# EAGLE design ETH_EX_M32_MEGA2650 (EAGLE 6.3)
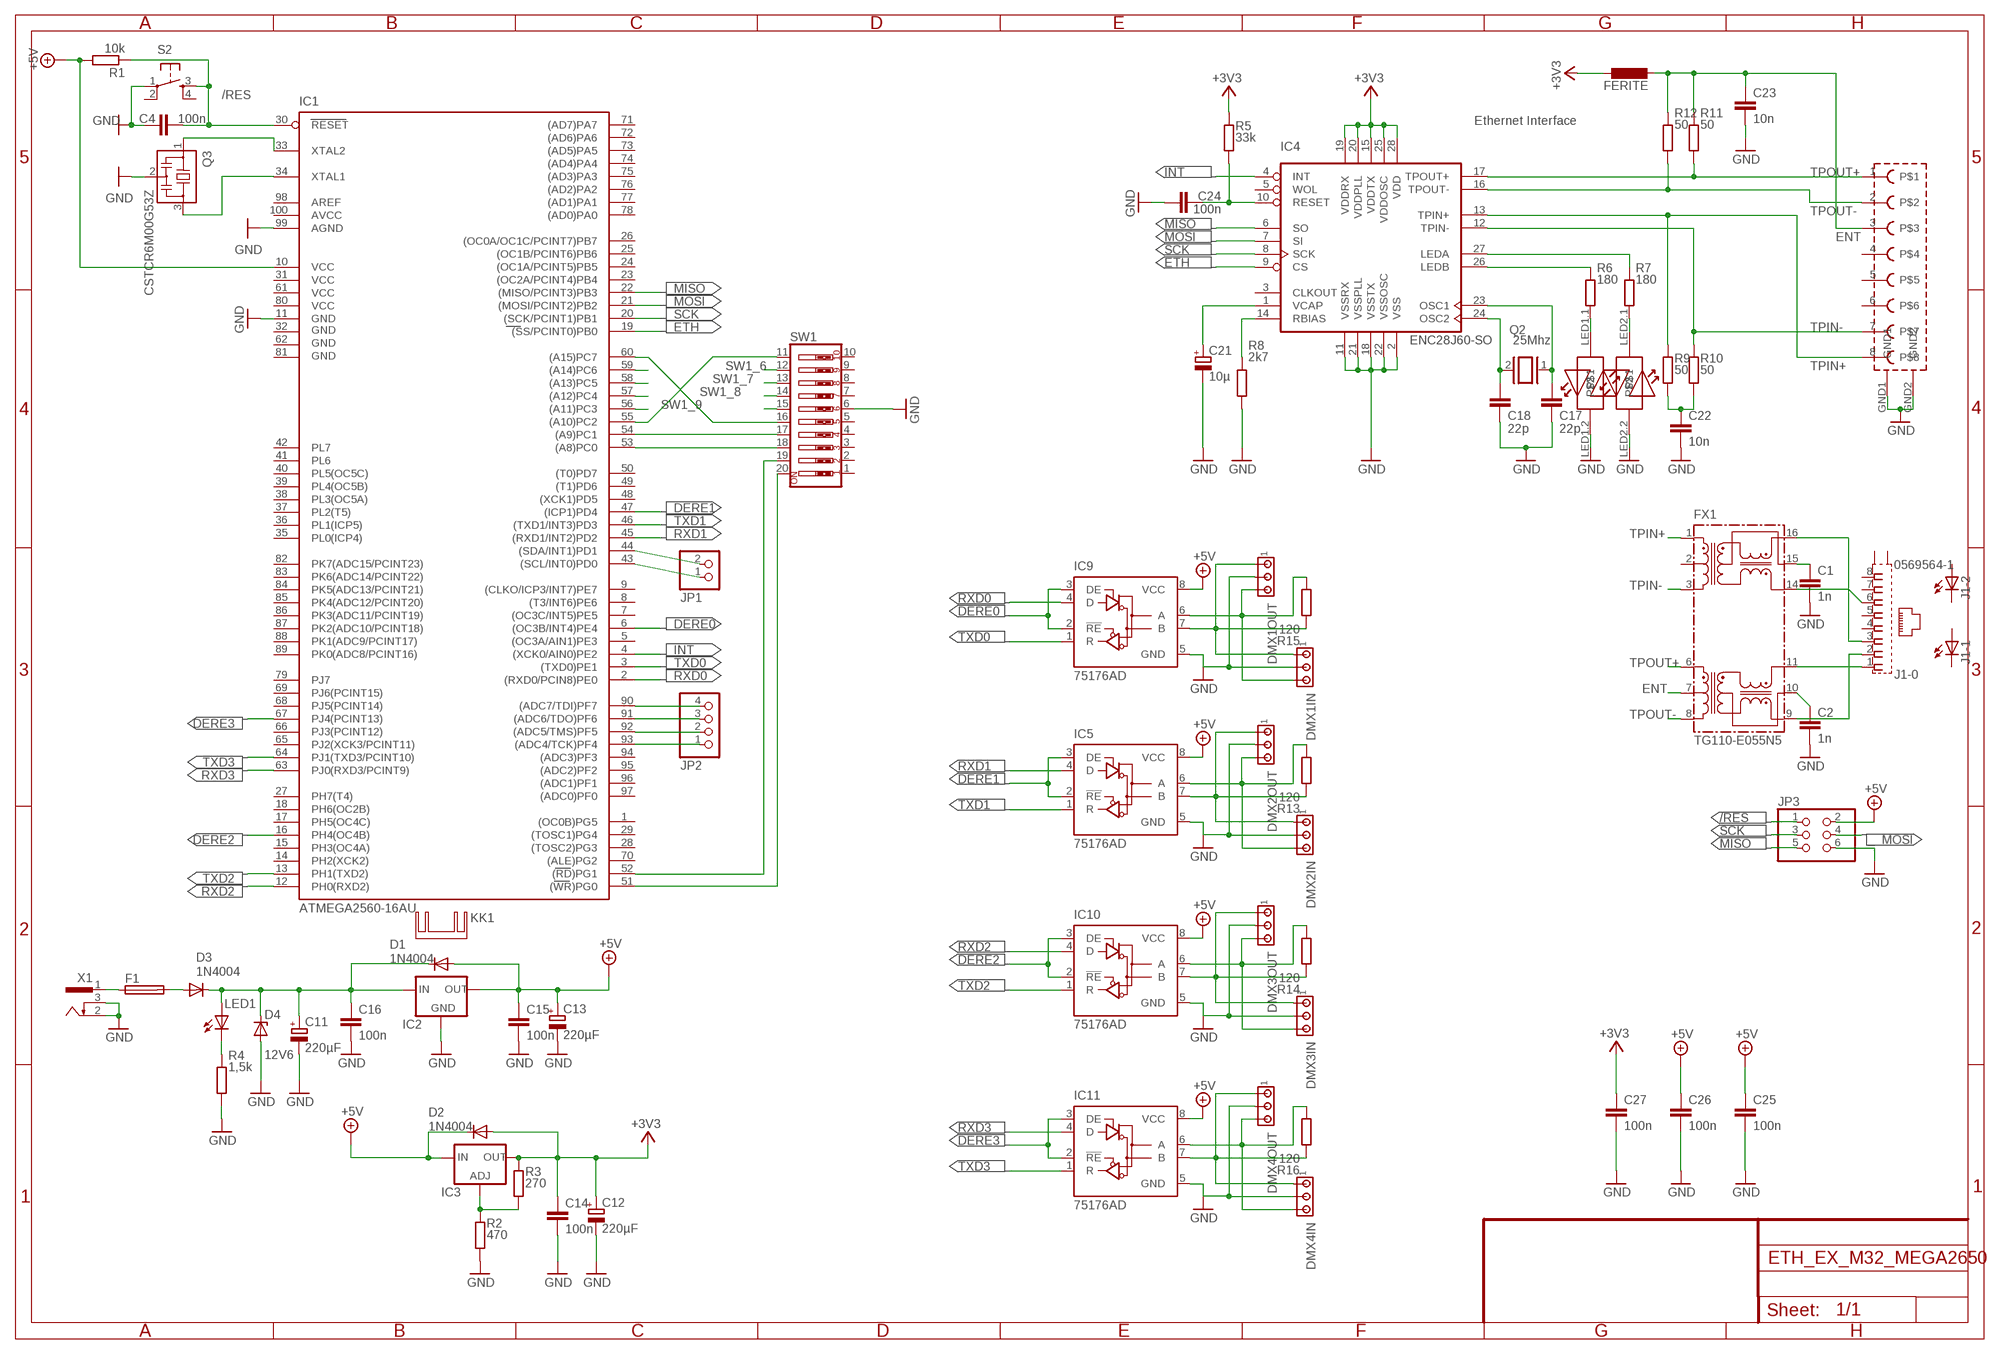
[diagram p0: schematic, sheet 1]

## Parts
C1  1n  C-EUC0805K  [C0805K]
C2  1n  C-EUC0805K  [C0805K]
C4  100n  C-EUC0805K  [C0805K]
C11  220µF  CPOL-EUE3.5-8  [E3,5-8]
C12  220µF  CPOL-EUE3.5-8  [E3,5-8]
C13  220µF  CPOL-EUE3.5-8  [E3,5-8]
C14  100n  C-EU025-024X044  [C025-024X044]
C15  100n  C-EU050-024X044  [C050-024X044]
C16  100n  C-EU050-024X044  [C050-024X044]
C17  22p  C-EUC0805K  [C0805K]
C18  22p  C-EUC0805K  [C0805K]
C21  10µ  CPOL-EUD  [PANASONIC_D]
C22  10n  C-EUC0805K  [C0805K]
C23  10n  C-EUC0805K  [C0805K]
C24  100n  C-EUC0805K  [C0805K]
C25  100n  C-EUC0805K  [C0805K]
C26  100n  C-EUC0805K  [C0805K]
C27  100n  C-EUC0805K  [C0805K]
D1  1N4004  [DO41-10]
D2  1N4004  [DO41-10]
D3  1N4004  [DO41-10]
D4  12V6  BZX90  [DO34Z7]
DMX1IN  MTA03-100  [10X03MTA]
DMX1OUT  MTA03-100  [10X03MTA]
DMX2IN  MTA03-100  [10X03MTA]
DMX2OUT  MTA03-100  [10X03MTA]
DMX3IN  MTA03-100  [10X03MTA]
DMX3OUT  MTA03-100  [10X03MTA]
DMX4IN  MTA03-100  [10X03MTA]
DMX4OUT  MTA03-100  [10X03MTA]
F1  PICOFUSE  [PICOFUSE]
FERITE  L-EU0204/5  [0204/5@1]
FX1  TG110-E055N5  [N5]
IC1  ATMEGA2560-16AU  [TQFP100]
IC2  78XXS  [78XXS]
IC3  LM317TS  [317TS]
IC4  ENC28J60-SO  [SO28W]
IC5  75176AD  [D_R-PDSO-G8]
IC9  75176AD  [D_R-PDSO-G8]
IC10  75176AD  [D_R-PDSO-G8]
IC11  75176AD  [D_R-PDSO-G8]
J1  0569564-1  [0569564]
JP1  PINHD-1X2_2.54  [1X02]
JP2  PINHD-1X4_2.54  [1X04]
JP3  PINHD-2X3_2.54-SMD  [2X03SMD]
KK1  SK95-2M3  [SK95-2M3]
LED1  LED3MM  [LED3MM]
Q2  25Mhz  XTAL/S  [QS]
Q3  CSTCR6M00G53Z  [CSTCR6M]
R1  10k  R-EU_R0805  [R0805]
R2  470  R-EU_0207/10  [0207/10]
R3  270  R-EU_0207/10  [0207/10]
R4  1,5k  R-EU_0207/10  [0207/10]
R5  33k  R-EU_R0805  [R0805]
R6  180  R-EU_R0805  [R0805]
R7  180  R-EU_R0805  [R0805]
R8  2k7  R-EU_R0805  [R0805]
R9  50  R-EU_R0805  [R0805]
R10  50  R-EU_R0805  [R0805]
R11  50  R-EU_R0805  [R0805]
R12  50  R-EU_R0805  [R0805]
R13  120  R-EU_R0805  [R0805]
R14  120  R-EU_R0805  [R0805]
R15  120  R-EU_R0805  [R0805]
R16  120  R-EU_R0805  [R0805]
S2  TASTER_93XX  [TASTER_93XX]
SW1  SW_DIP-10  [EDG-10]
U$1  MAGJACK  [MAGJACK]
X1  SCD-014A  [SCD-014-A]

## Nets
+3V3: C12.+ C14.1 C27.1 D2.A FERITE.1 IC3.2(OUT) IC4.15(VDDTX) IC4.19(VDDRX) IC4.20(VDDPLL) IC4.25(VDDOSC) IC4.28(VDD) R3.2 R5.2
+5V: C13.+ C15.1 C25.2 C26.1 D1.A IC1.10(VCC) IC2.OUT IC5.8(VCC) IC9.8(VCC) IC10.8(VCC) IC11.8(VCC) JP3.2 R1.2
/RES: C4.2 IC1.30(RESET) JP3.1 R1.1 S2.3(S)
DERE0: IC1.6((OC3B/INT4)PE4) IC9.2(!RE) IC9.3(DE)
DERE1: IC1.47((ICP1)PD4) IC5.2(!RE) IC5.3(DE)
DERE2: IC1.16(PH4(OC4B)) IC10.2(!RE) IC10.3(DE)
DERE3: IC1.67(PJ4(PCINT13)) IC11.2(!RE) IC11.3(DE)
ENT: C23.1 FERITE.2 FX1.7 R11.1 R12.1 U$1.3
ETH: IC1.19((SS/PCINT0)PB0) IC4.9(CS)
GND: C1.2 C2.2 C4.1 C11.- C12.- C13.- C14.2 C15.2 C16.2 C17.1 C18.1 C21.- C22.2 C23.2 C24.1 C25.1 C26.2 C27.2 D4.A DMX1IN.2 DMX1OUT.2 DMX2IN.2 DMX2OUT.2 DMX3IN.2 DMX3OUT.2 DMX4IN.2 DMX4OUT.2 IC1.11(GND) IC1.99(AGND) IC2.GND IC4.2(VSS) IC4.11(VSSRX) IC4.18(VSSTX) IC4.21(VSSPLL) IC4.22(VSSOSC) IC5.5(GND) IC9.5(GND) IC10.5(GND) IC11.5(GND) JP3.6 Q3.2 R2.1 R4.1 R8.1 S2.1(P) SW1.6 U$1.GND1 U$1.GND2 U$1.LED1.2 U$1.LED2.2 X1.2 X1.3
INT: IC1.4((XCK0/AIN0)PE2) IC4.4(INT)
MISO: IC1.22((MISO/PCINT3)PB3) IC4.6(SO) JP3.5
MOSI: IC1.21((MOSI/PCINT2)PB2) IC4.7(SI) JP3.4
N$1: IC1.34(XTAL1) Q3.3
N$2: IC1.33(XTAL2) Q3.1
N$3: IC1.51((WR)PG0) SW1.20
N$4: LED1.K(C) R4.2
N$5: IC1.52((RD)PG1) SW1.19
N$6: D3.A F1.2
N$7: IC1.53((A8)PC0) SW1.18
N$8: R7.1 U$1.LED2.1
N$9: IC1.54((A9)PC1) SW1.17
N$10: F1.1 X1.1
N$11: IC4.27(LEDA) R7.2
N$12: IC3.1(ADJ) R2.2 R3.1
N$13: IC4.26(LEDB) R6.2
N$14: R6.1 U$1.LED1.1
N$15: DMX2IN.1 DMX2OUT.1 IC5.7(B) R13.2
N$16: DMX2IN.3 DMX2OUT.3 IC5.6(A) R13.1
N$17: DMX1IN.3 DMX1OUT.3 IC9.6(A) R15.1
N$18: DMX3IN.1 DMX3OUT.1 IC10.7(B) R14.2
N$19: DMX3IN.3 DMX3OUT.3 IC10.6(A) R14.1
N$20: C18.2 IC4.24(OSC2) Q2.2
N$21: C17.2 IC4.23(OSC1) Q2.1
N$26: IC4.14(RBIAS) R8.2
N$27: C21.+ IC4.1(VCAP)
N$28: DMX4IN.1 DMX4OUT.1 IC11.7(B) R16.2
N$29: C22.1 R9.1 R10.1
N$30: C24.2 IC4.10(RESET) R5.1
N$31: DMX1IN.1 DMX1OUT.1 IC9.7(B) R15.2
N$32: DMX4IN.3 DMX4OUT.3 IC11.6(A) R16.1
N$33: FX1.11 J1.1
N$34: FX1.9 J1.2
N$35: FX1.16 J1.3
N$36: FX1.14 J1.6
N$37: IC1.90((ADC7/TDI)PF7) JP2.4
N$38: IC1.91((ADC6/TDO)PF6) JP2.3
N$39: IC1.92((ADC5/TMS)PF5) JP2.2
N$40: IC1.93((ADC4/TCK)PF4) JP2.1
N$41: IC1.43((SCL/INT0)PD0) JP1.1
N$42: IC1.44((SDA/INT1)PD1) JP1.2
N$43: C2.1 FX1.10
N$44: C1.1 FX1.15
N$250: C11.+ C16.1 D1.C D3.C D4.C IC2.IN LED1.A
RXD0: IC1.2((RXD0/PCIN8)PE0)
RXD1: IC1.45((RXD1/INT2)PD2) IC5.4(D)
RXD2: IC1.12(PH0(RXD2)) IC10.4(D)
RXD3: IC1.63(PJ0(RXD3/PCINT9)) IC11.4(D)
SCK: IC1.20((SCK/PCINT1)PB1) IC4.8(SCK) JP3.3
SW1_5: IC1.60((A15)PC7) SW1.16
SW1_6: IC1.59((A14)PC6) SW1.15
SW1_7: IC1.58((A13)PC5) SW1.14
SW1_8: IC1.57((A12)PC4) SW1.13
SW1_9: IC1.56((A11)PC3) SW1.12
SW1_10: IC1.55((A10)PC2) SW1.11
TPIN+: FX1.1 IC4.13(TPIN+) R9.2 U$1.8
TPIN-: FX1.3 IC4.12(TPIN-) R10.2 U$1.7
TPOUT+: FX1.6 IC4.17(TPOUT+) R11.2 U$1.1
TPOUT-: FX1.8 IC4.16(TPOUT-) R12.2 U$1.2
TXD0: IC1.3((TXD0)PE1) IC9.1(R)
TXD1: IC1.46((TXD1/INT3)PD3) IC5.1(R)
TXD2: IC1.13(PH1(TXD2)) IC10.1(R)
TXD3: IC1.64(PJ1(TXD3/PCINT10)) IC11.1(R)
VCC: D2.C IC3.3(IN) ; supply symbol labelled +5V
Unconnected: FX1.2 IC1.1((OC0B)PG5) IC1.5((OC3A/AIN1)PE3) IC1.7((OC3C/INT5)PE5) IC1.8((T3/INT6)PE6) IC1.9((CLKO/ICP3/INT7)PE7) IC1.14(PH2(XCK2)) IC1.15(PH3(OC4A)) IC1.17(PH5(OC4C)) IC1.18(PH6(OC2B)) IC1.23((OC2A/PCINT4)PB4) IC1.24((OC1A/PCINT5)PB5) IC1.25((OC1B/PCINT6)PB6) IC1.26((OC0A/OC1C/PCINT7)PB7) IC1.27(PH7(T4)) IC1.28((TOSC2)PG3) IC1.29((TOSC1)PG4) IC1.35(PL0(ICP4)) IC1.36(PL1(ICP5)) IC1.37(PL2(T5)) IC1.38(PL3(OC5A)) IC1.39(PL4(OC5B)) IC1.40(PL5(OC5C)) IC1.41(PL6) IC1.42(PL7) IC1.48((XCK1)PD5) IC1.49((T1)PD6) IC1.50((T0)PD7) IC1.65(PJ2(XCK3/PCINT11)) IC1.66(PJ3(PCINT12)) IC1.68(PJ5(PCINT14)) IC1.69(PJ6(PCINT15)) IC1.70((ALE)PG2) IC1.71((AD7)PA7) IC1.72((AD6)PA6) IC1.73((AD5)PA5) IC1.74((AD4)PA4) IC1.75((AD3)PA3) IC1.76((AD2)PA2) IC1.77((AD1)PA1) IC1.78((AD0)PA0) IC1.79(PJ7) IC1.82(PK7(ADC15/PCINT23)) IC1.83(PK6(ADC14/PCINT22)) IC1.84(PK5(ADC13/PCINT21)) IC1.85(PK4(ADC12/PCINT20)) IC1.86(PK3(ADC11/PCINT19)) IC1.87(PK2(ADC10/PCINT18)) IC1.88(PK1(ADC9/PCINT17)) IC1.89(PK0(ADC8/PCINT16)) IC1.94((ADC3)PF3) IC1.95((ADC2)PF2) IC1.96((ADC1)PF1) IC1.97((ADC0)PF0) IC1.98(AREF) IC4.3(CLKOUT) IC4.5(WOL) IC9.4(D) J1.4 J1.5 J1.7 J1.8 J1.A1(-1:A) J1.A2(-2:A) J1.C1(-1:C) J1.C2(-2:C) J1.S1(-0:S1) J1.S2(-0:S2) S2.2(P1) S2.4(S1) SW1.1 SW1.2 SW1.3 SW1.4 SW1.5 SW1.7 SW1.8 SW1.9 SW1.10 U$1.4 U$1.5 U$1.6

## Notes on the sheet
- Ethernet Interface

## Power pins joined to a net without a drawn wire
AVCC: IC1.100(AVCC)
GND1: IC1.32(GND1)
GND2: IC1.62(GND2)
GND3: IC1.81(GND3)
VCC1: IC1.31(VCC1)
VCC2: IC1.61(VCC2)
VCC3: IC1.80(VCC3)

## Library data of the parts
C1 C2 C4 C17 C18 C22-C27 = resistor:C-EU: CAPACITOR, European symbol
C11-C13 = rcl:CPOL-EU: POLARIZED CAPACITOR, European symbol
C14-C16 = rcl:C-EU: CAPACITOR, European symbol
C21 = resistor:CPOL-EU: POLARIZED CAPACITOR, European symbol
D1-D3 = diode:1N4004: DIODE
D4 = diode:BZX90: Z DIODE
DMX1IN DMX1OUT DMX2IN DMX2OUT DMX3IN DMX3OUT DMX4IN DMX4OUT = con-amp:MTA03-100: AMP connector
F1 = fuse:PICOFUSE: PICOFUSE
FERITE = rcl:L-EU: INDUCTOR, European symbol
FX1 = halo-electronics:TG110-E*N5: E-Ultra (TM) 10/100BASE-TX SOIC-16 Fast Ethernet Magnetic Modules Source: www.haloelectronics.com .. e-ultra.pdf
IC1 = atmel-2005:ATMEGA*: MICROCONTROLLER 64/128/256 Kbytes FLASH 4 Kbytes EEPROM 8 Kbytes SRAM 86 General Purpose I/O pins 12-channels16-bit PWM 4 x Serial USARTs 16-channels 10-bit A/D
IC2 = v-reg:78XXS: VOLTAGE REGULATOR
IC3 = v-reg:LM317TS: VOLTAGE REGULATOR
IC4 = enc28j60centered:ENC28J60-*: Microchip 10Mbit Ethernet controller with SPI interface Improved SOIC28 layout (pads in 0.01 raster, pin1 slightly smaller). Pin 6 (SO) changed from Out (paralleling several Outs gives an error) to OC. Author: Profi from mikrocontroller.net - forum Date: 2006.0827
IC5 IC9-IC11 = 751xx:75176A: DIFFERENTIAL BUS TRANSCEIVER Source: http://focus.ti.com/lit/ds/symlink/sn75176a.pdf
J1 = con-amp:0569564-*: MODULAR JACK 8 POS., RIGHT ANGLE, LOW PROFILE WITH LEDS Source: http://ecommas.tycoelectronics.com/.. 569564_K.pdf
JP1 = pinhead-1:PINHD-1X2: PIN HEADER
JP2 = pinhead-1:PINHD-1X4: PIN HEADER
JP3 = pinhead-1:PINHD-2X3: PIN HEADER
KK1 = heatsink:SK95-2M3: HEATSINK
LED1 = led:LED: LED
Q2 = special:XTAL/S: CRYSTAL
Q3 = murata-filter:CSTCR: Resonator Source: murata.co.jp; MPN: CSTCR6M00G53-R0; OC_FARNELL: 1170434; OC_NEWARK: 25M8759
R1 R5-R16 = resistor:R-EU_: RESISTOR, European symbol
R2-R4 = rcl:R-EU_: RESISTOR, European symbol
S2 = uwegw:TASTER_93XX: OMRON SWITCH
SW1 = special:SW_DIP-10: DIP SWITCH
U$1 = magjacksmalldrill:MAGJACK
X1 = con-shiua-chyuan:SCD-014A: Power Jack 2.5mm

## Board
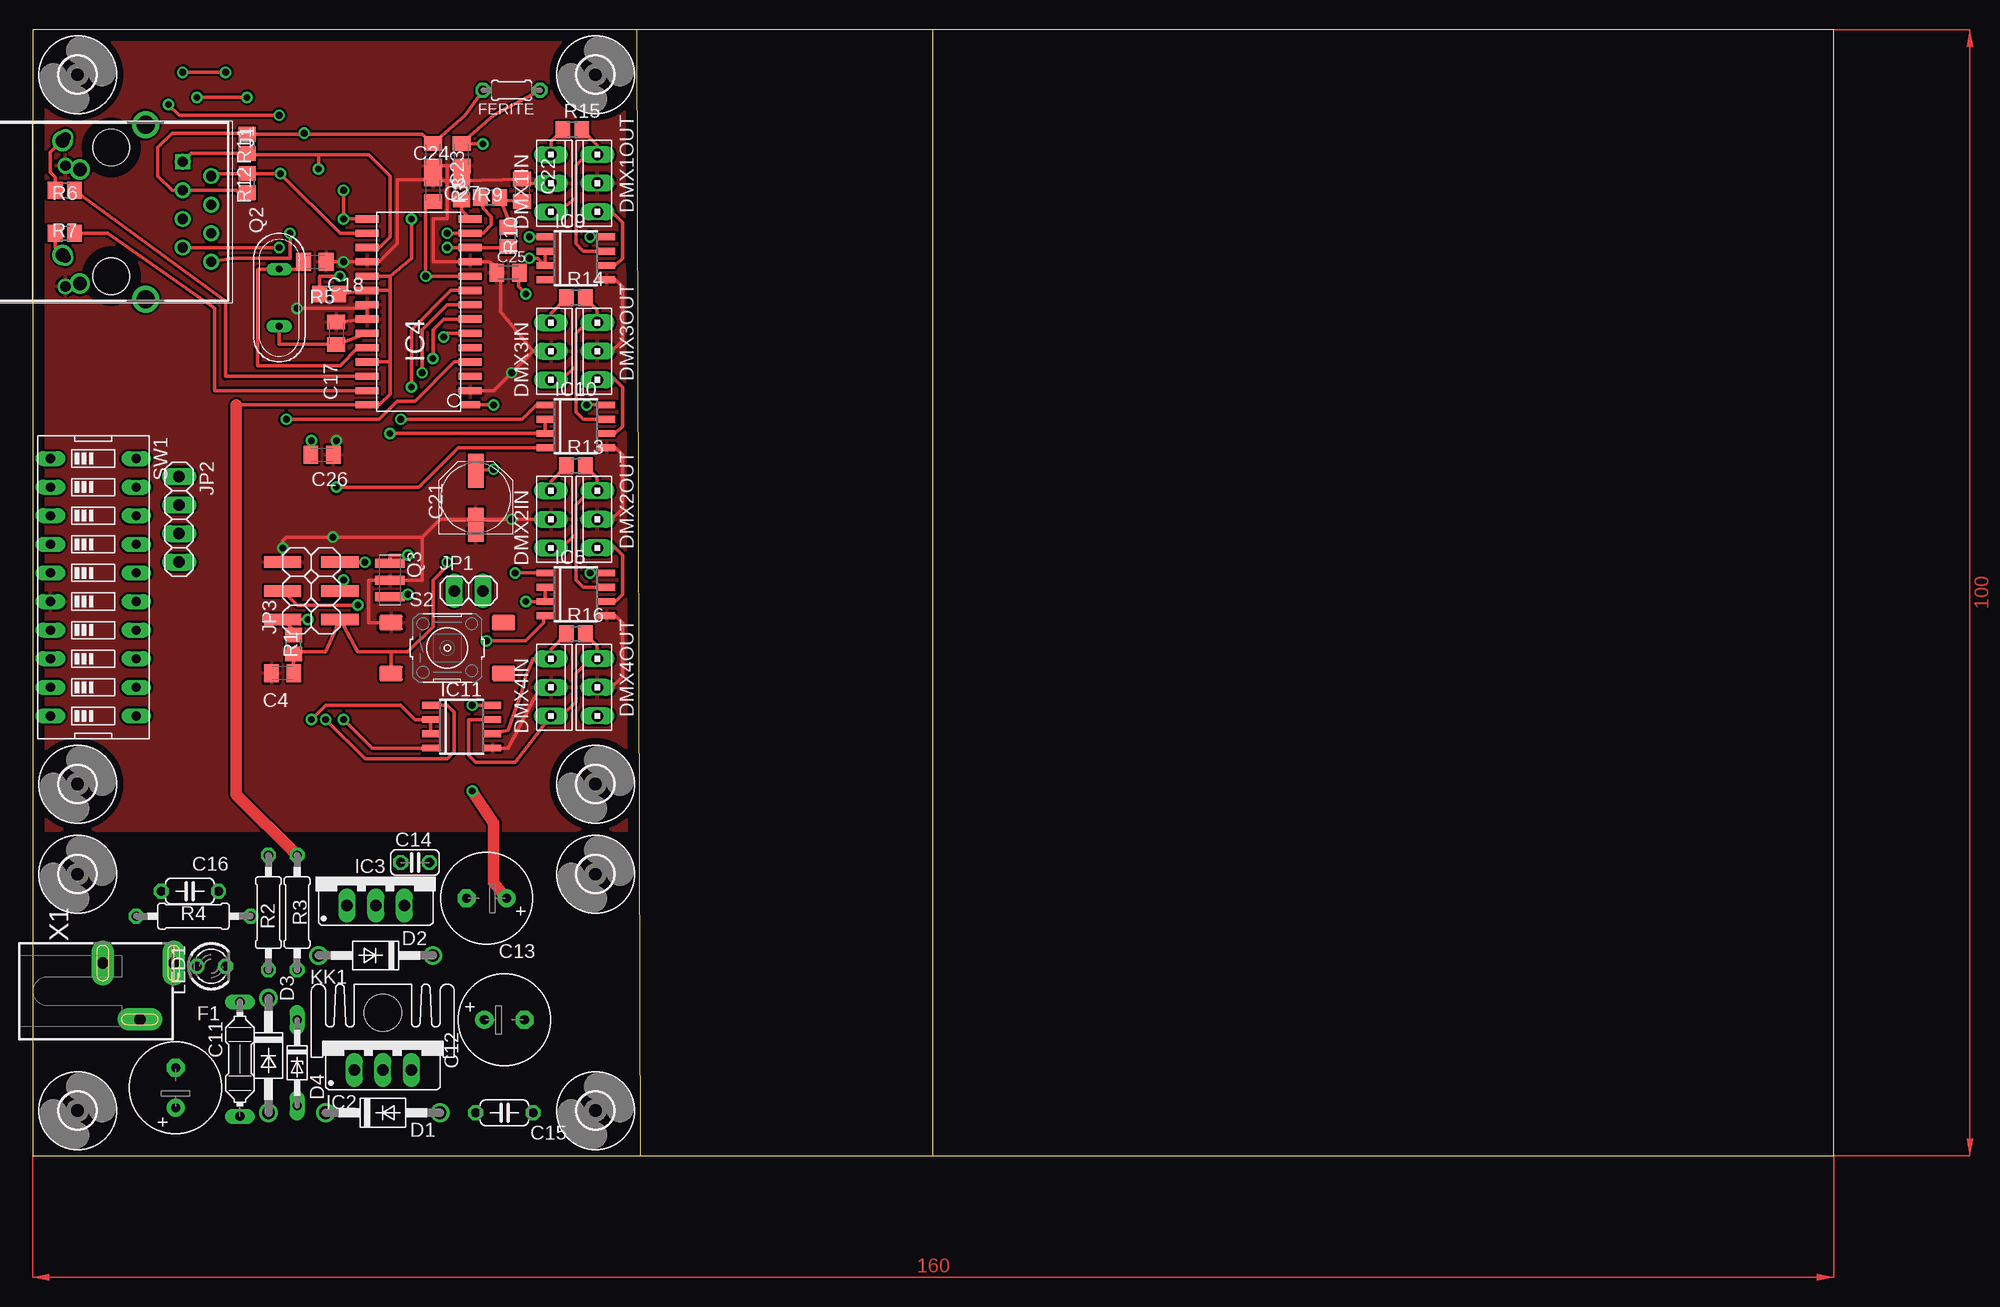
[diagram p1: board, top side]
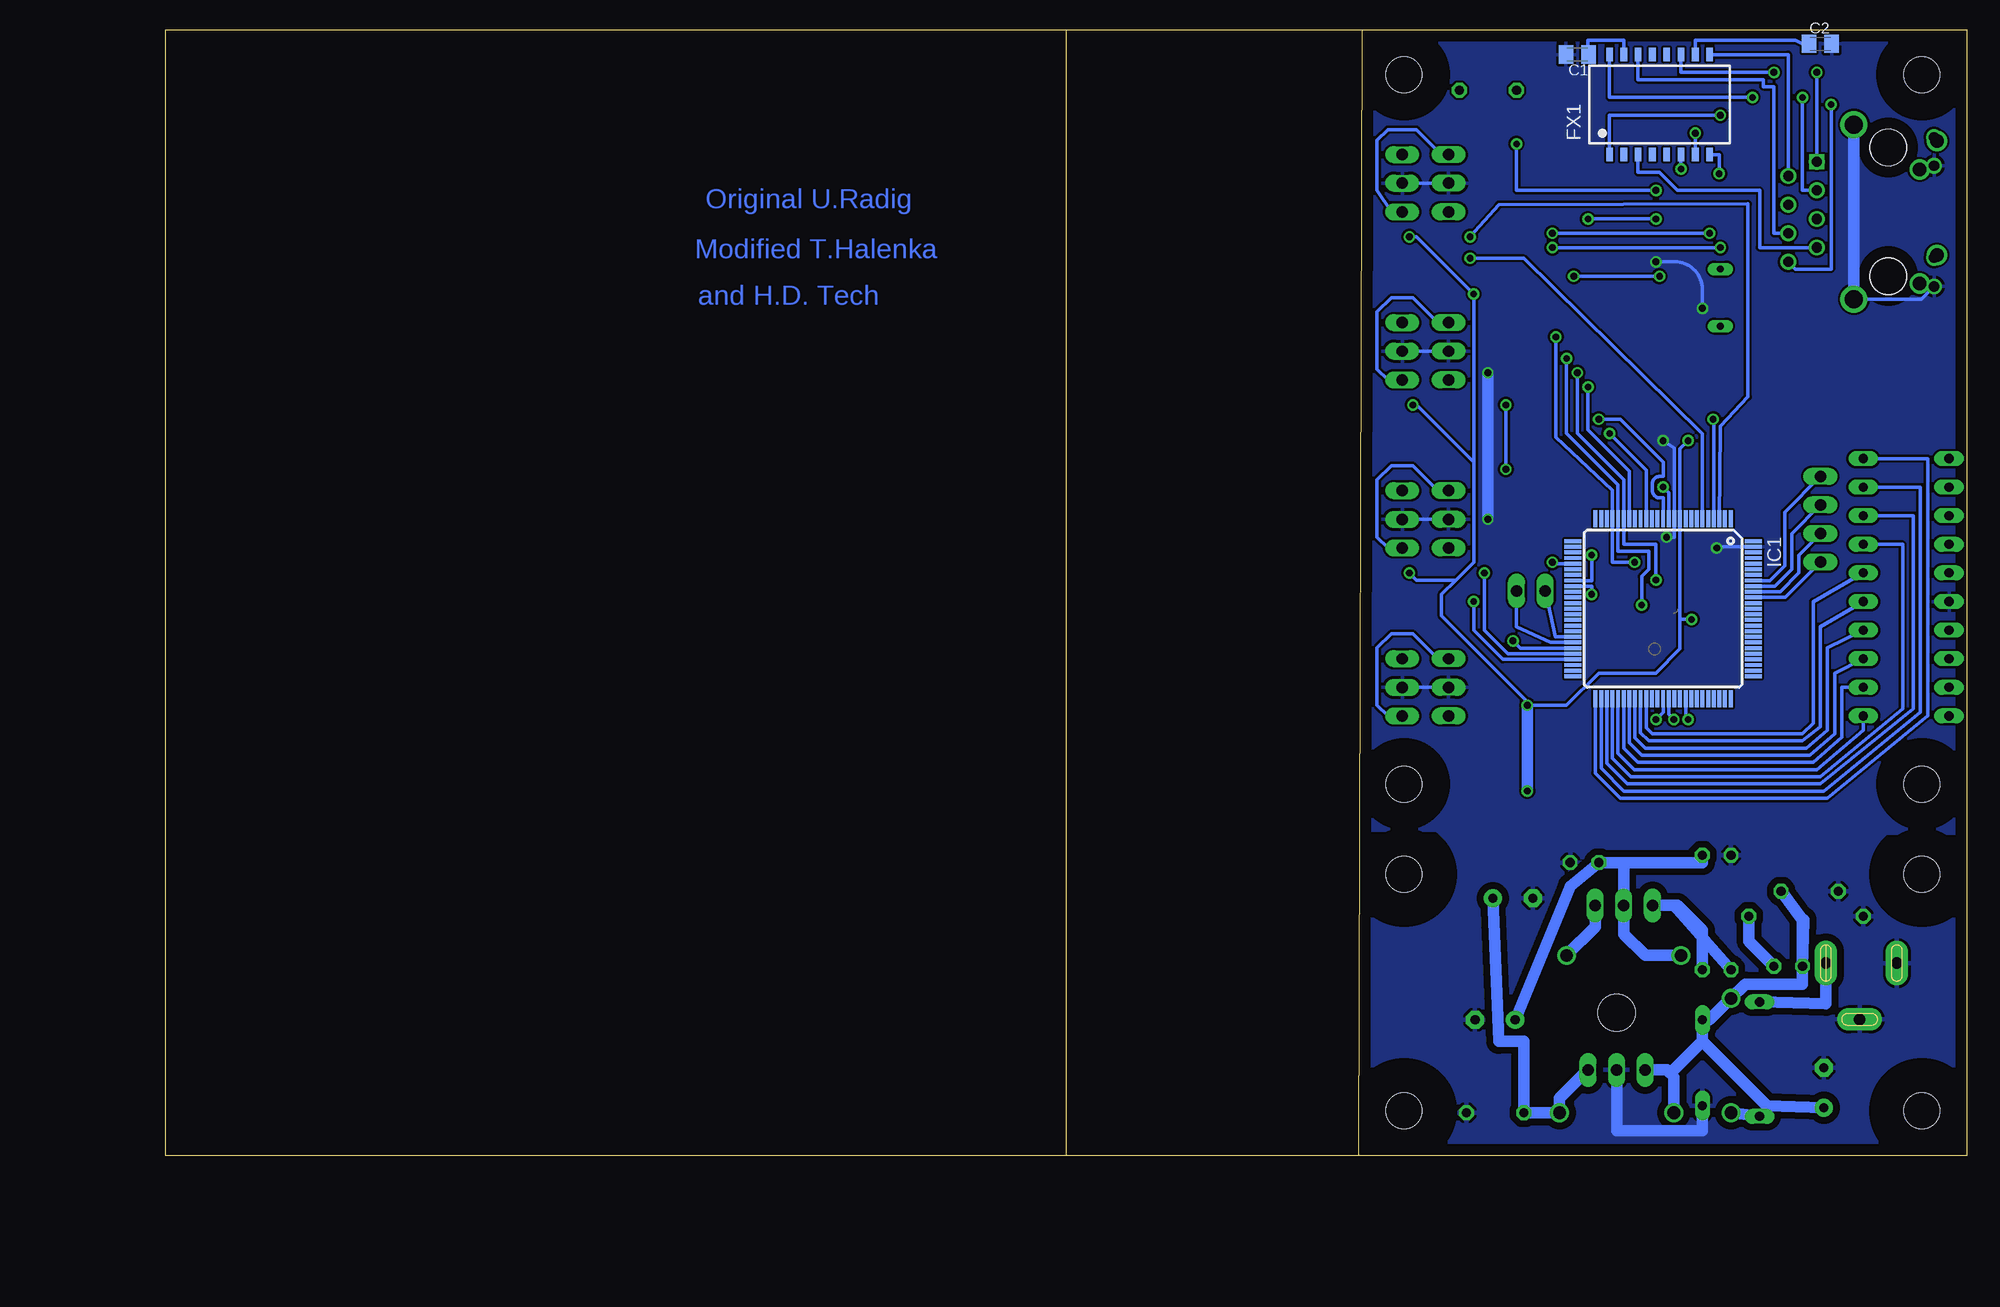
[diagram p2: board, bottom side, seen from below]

Size 160 x 100 mm. Coordinates in mm from the lower left corner, seen from the top.
Outline: 54,0 0,0 0,100 53.68,100
Outline: 54,0 80,0
Outline: 80,0 160,0 160,100 80,100
Outline: 80,100 53.68,100
Outline: 80,0 80,100
Outline: 54,0 53.68,100
Copper layers (1*16): Top 0.035mm / dielectric 1.5mm / Bottom 0.035mm
Design rules "default": minimum track width 10mil, minimum drill 24mil, track to track 8mil, track to pad 8mil, pad to pad 8mil, via to via 8mil, smd to smd 8mil, copper to edge 40mil, drill to drill 8mil, minimum pad ring 10mil, minimum via ring 8mil, stop-mask expansion 4mil, vias tented up to drill 0mil, thermal gap 10mil

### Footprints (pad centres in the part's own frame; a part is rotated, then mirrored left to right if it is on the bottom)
C0805K = smd 1.3 x 1.6: 1 -1,0; 2 1,0
E3,5-8 = drill 0.813 pad 1.6: + -1.778,0 | drill 0.813 pad 1.6 octagon: - 1.778,0
C025-024X044 = drill 0.813 octagon: 1 -1.27,0; 2 1.27,0
C050-024X044 = drill 0.813 octagon: 1 -2.54,0; 2 2.54,0
PANASONIC_D = smd 3 x 1.4: + 2.4,0; - -2.4,0
DO41-10 = drill 1.118: A 5.08,0; C -5.08,0
DO34Z7 = drill 0.813 long: A 3.81,0; C -3.81,0
10X03MTA = drill 1.016 long: 1 2.54,0; 2 0,0; 3 -2.54,0
PICOFUSE = drill 0.813 long: 1 -5.08,0; 2 5.08,0
0204/5@1 = drill 0.813 octagon: 1 -2.54,0; 2 2.54,0
N5 = smd 0.6 x 1.2: 1 -4.445,-4.445; 2 -3.175,-4.445; 3 -1.905,-4.445; 4 -0.635,-4.445; 5 0.635,-4.445; 6 1.905,-4.445; 7 3.175,-4.445; 8 4.445,-4.445; 9 4.445,4.445; 10 3.175,4.445; 11 1.905,4.445; 12 0.635,4.445; 13 -0.635,4.445; 14 -1.905,4.445; 15 -3.175,4.445; 16 -4.445,4.445
TQFP100 = smd 1.5 x 0.35: 1 -8,6; 2 -8,5.5; 3 -8,5; 4 -8,4.5; 5 -8,4; 6 -8,3.5; 7 -8,3; 8 -8,2.5; 9 -8,2; 10 -8,1.5; 11 -8,1; 12 -8,0.5; 13 -8,0; 14 -8,-0.5; 15 -8,-1; 16 -8,-1.5; 17 -8,-2; 18 -8,-2.5; 19 -8,-3; 20 -8,-3.5; 21 -8,-4; 22 -8,-4.5; 23 -8,-5; 24 -8,-5.5; 25 -8,-6; 51 8,-6; 52 8,-5.5; 53 8,-5; 54 8,-4.5; 55 8,-4; 56 8,-3.5; 57 8,-3; 58 8,-2.5; 59 8,-2; 60 8,-1.5; 61 8,-1; 62 8,-0.5; 63 8,0; 64 8,0.5; 65 8,1; 66 8,1.5; 67 8,2; 68 8,2.5; 69 8,3; 70 8,3.5; 71 8,4; 72 8,4.5; 73 8,5; 74 8,5.5; 75 8,6 | smd 0.35 x 1.5: 26 -6,-8; 27 -5.5,-8; 28 -5,-8; 29 -4.5,-8; 30 -4,-8; 31 -3.5,-8; 32 -3,-8; 33 -2.5,-8; 34 -2,-8; 35 -1.5,-8; 36 -1,-8; 37 -0.5,-8; 38 0,-8; 39 0.5,-8; 40 1,-8; 41 1.5,-8; 42 2,-8; 43 2.5,-8; 44 3,-8; 45 3.5,-8; 46 4,-8; 47 4.5,-8; 48 5,-8; 49 5.5,-8; 50 6,-8; 76 6,8; 77 5.5,8; 78 5,8; 79 4.5,8; 80 4,8; 81 3.5,8; 82 3,8; 83 2.5,8; 84 2,8; 85 1.5,8; 86 1,8; 87 0.5,8; 88 0,8; 89 -0.5,8; 90 -1,8; 91 -1.5,8; 92 -2,8; 93 -2.5,8; 94 -3,8; 95 -3.5,8; 96 -4,8; 97 -4.5,8; 98 -5,8; 99 -5.5,8; 100 -6,8
78XXS = drill 1.016 long: GND 0,-2.54; IN -2.54,-2.54; OUT 2.54,-2.54
317TS = drill 1.016 long: 1 -2.54,-2.54; 2 0,-2.54; 3 2.54,-2.54
SO28W = smd 0.635 x 1.778: 1 -8.255,-4.572 | smd 0.635 x 2.032: 2 -6.985,-4.572; 3 -5.715,-4.572; 4 -4.445,-4.572; 5 -3.175,-4.572; 6 -1.905,-4.572; 7 -0.635,-4.572; 8 0.635,-4.572; 9 1.905,-4.572; 10 3.175,-4.572; 11 4.445,-4.572; 12 5.715,-4.572; 13 6.985,-4.572; 14 8.255,-4.572; 15 8.255,4.572; 16 6.985,4.572; 17 5.715,4.572; 18 4.445,4.572; 19 3.175,4.572; 20 1.905,4.572; 21 0.635,4.572; 22 -0.635,4.572; 23 -1.905,4.572; 24 -3.175,4.572; 25 -4.445,4.572; 26 -5.715,4.572; 27 -6.985,4.572; 28 -8.255,4.572
D_R-PDSO-G8 = smd 0.6 x 1.5: 1 -1.905,-2.75; 2 -0.635,-2.75; 3 0.635,-2.75; 4 1.905,-2.75; 5 1.905,2.75; 6 0.635,2.75; 7 -0.635,2.75; 8 -1.905,2.75
0569564 = drill 0.9: 1 -4.445,6.35; 2 -3.175,8.89; 3 -1.905,6.35; 4 -0.635,8.89; 5 0.635,6.35; 6 1.905,8.89; 7 3.175,6.35; 8 4.445,8.89 | drill 1.2: A1 -6.295,-4.32; A2 3.835,-4.32; C1 -3.755,-2.79; C2 6.375,-2.79 | drill 1.6: S1 -7.745,3.05; S2 7.745,3.05 | hole 3.25: -5.715,0; 5.715,0
1X02 = drill 1.016 long: 1 -1.27,0; 2 1.27,0
1X04 = drill 1.016 long: 1 -3.81,0; 2 -1.27,0; 3 1.27,0; 4 3.81,0
2X03SMD = smd 1.016 x 3.302: 1 -1.27,-3.81; 2 -1.27,1.27; 3 1.27,-3.81; 4 1.27,1.27; 5 3.81,-3.81; 6 3.81,1.27
SK95-2M3 = hole 3.302: 0,2.54
LED3MM = drill 0.813 octagon: A -1.27,0; K 1.27,0
QS = drill 0.61 long: 1 -2.54,0; 2 2.54,0
CSTCR6M = smd 0.8 x 2.6: 1 -1.5,0; 2 0,0; 3 1.5,0
R0805 = smd 1.3 x 1.5: 1 -0.85,0; 2 0.85,0
0207/10 = drill 0.813 octagon: 1 -5.08,0; 2 5.08,0
TASTER_93XX = smd 2.1 x 1.4: 1 -5,2.25; 2 5,2.25; 3 -5,-2.25; 4 5,-2.25
EDG-10 = drill 0.813 long: 1 -11.43,-3.81; 2 -8.89,-3.81; 3 -6.35,-3.81; 4 -3.81,-3.81; 5 -1.27,-3.81; 6 1.27,-3.81; 7 3.81,-3.81; 8 6.35,-3.81; 9 8.89,-3.81; 10 11.43,-3.81; 11 11.43,3.81; 12 8.89,3.81; 13 6.35,3.81; 14 3.81,3.81; 15 1.27,3.81; 16 -1.27,3.81; 17 -3.81,3.81; 18 -6.35,3.81; 19 -8.89,3.81; 20 -11.43,3.81
MAGJACK = drill 0.8 square: 1 -4.445,6.35 | drill 0.8: 2 -3.175,8.89; 3 -1.905,6.35; 4 -0.635,8.89; 5 0.635,6.35; 6 1.905,8.89; 7 3.175,6.35; 8 4.445,8.89 | drill 1.3: GND1 -7.747,3.048; GND2 7.747,3.048 | drill 0.9: LED1.1 -6.629,-4.064; LED1.2 -4.089,-4.064; LED2.1 4.089,-4.064; LED2.2 6.629,-4.064 | hole 3.2: -5.715,0; 5.715,0
3,2 = hole 3.2: 0,0
SCD-014-A = drill 1 pad 2 long: 1 -2.5,13.8; 2 -2.5,7.5; 3 2.5,10.8

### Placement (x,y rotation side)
C1  34.61,97.79 180 bottom
C2  13.02,98.74 0 bottom
C4  22.23,42.86 0 top
C11  12.7,6.03 90 top
C12  41.91,12.06 0 top
C13  40.32,22.86 180 top
C14  33.97,26.04 0 top
C15  41.91,3.81 0 top
C16  13.97,23.5 180 top
C17  26.99,73.03 270 top
C18  25.08,79.38 180 top
C21  39.37,58.42 90 top
C22  43.5,85.72 90 top
C23  35.56,88.9 270 top
C24  35.56,85.72 270 top
C25  42.23,78.42 0 top
C26  25.72,62.23 0 top
C27  38.1,88.9 270 top
D1  31.11,3.81 0 top
D2  30.48,17.78 180 top
D3  20.95,8.89 270 top
D4  23.5,8.26 270 top
DMX1IN  46.04,86.36 270 top
DMX1OUT  50.16,86.36 90 top
DMX2IN  46.04,56.52 270 top
DMX2OUT  50.16,56.52 90 top
DMX3IN  46.04,71.44 270 top
DMX3OUT  50.16,71.44 90 top
DMX4IN  46.04,41.59 270 top
DMX4OUT  50.16,41.59 90 top
F1  18.41,8.57 270 top
FERITE  42.55,94.61 180 top
FX1  27.3,93.34 0 bottom
IC1  26.99,48.58 270 bottom
IC2  31.11,10.16 0 top
IC3  30.48,24.77 0 top
IC4  34.29,74.93 90 top
IC5  48.26,49.85 270 top
IC9  48.26,79.69 270 top
IC10  48.26,64.77 270 top
IC11  38.1,38.1 270 top
J1  6.99,83.82 270 top
JP1  38.73,50.16 0 top
JP2  13.02,56.52 270 top
JP3  23.5,48.9 90 top
KK1  31.11,10.16 0 top
LED1  15.88,16.83 0 top
Q2  21.91,76.2 90 top
Q3  31.75,51.12 270 top
R1  23.18,45.4 90 top
R2  20.95,21.59 270 top
R3  23.5,21.59 90 top
R4  14.29,21.27 0 top
R5  26.35,76.52 0 top
R6  2.86,85.72 0 top
R7  2.86,81.92 0 top
R8  38.1,85.72 270 top
R9  40.64,85.09 180 top
R10  42.23,81.6 270 top
R11  19.05,89.85 270 top
R12  19.05,86.36 90 top
R13  48.26,61.28 0 top
R14  48.26,76.2 0 top
R15  47.94,91.12 0 top
R16  48.26,46.35 0 top
S2  36.83,45.09 0 top
SW1  5.4,50.48 270 top
U$1  6.99,83.82 270 top
U$2  [3,2]  4,4 0 top
U$5  [3,2]  4,25 0 top
U$6  [3,2]  50,25 0 top
U$7  [3,2]  50,4 0 top
U$8  [3,2]  4,33 0 top
U$9  [3,2]  50,33 0 top
U$10  [3,2]  4,96 0 top
U$11  [3,2]  50,96 0 top
X1  -1.27,14.61 270 top

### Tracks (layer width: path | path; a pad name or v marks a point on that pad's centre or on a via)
+3V3  (via drill 0.6)
  Top 0.305: R5.2 IC4.20 31.75,76.83 | 31.75,70.48 31.75,67.63 30.8,66.67 IC4.28 18.1,66.67 | 31.75,70.48 31.75,76.83 | 31.75,76.83 31.75,78.11 | 31.75,78.11 IC4.19 | IC4.25 31.75,70.48 | IC4.15 v27.62,83.19 v27.62,85.72 | v33.66,83.19 33.66,79.69 31.75,78.11 | v40.01,89.85 38.2,89.85 C27.1 40.96,92.39 FERITE.1
  Top 1.016: R3.2 18.1,32.07 18.1,66.67
  Bottom 0.305: v27.62,83.19 v33.66,83.19 | v40.01,89.85 40.01,85.72 v27.62,85.72
  Bottom 1.016: D2.A 28.57,17.78 30.48,19.68 IC3.2 30.48,26.04 | R3.2 23.5,26.04 30.48,26.04 | 30.48,26.04 C14.1 35.24,23.94 C12.+
+5V  (via drill 0.6)
  Top 0.305: v24.77,63.5 24.77,62.27 C26.1 | v24.45,47.62 JP3.2 23.18,46.67 R1.2 | IC9.8 v49.53,81.6 | v49.53,51.75 IC5.8 | IC11.8 v39.05,40.01 | IC10.8 v49.21,66.67 | v43.81,76.52 43.18,77.15 C25.2
  Top 1.016: v39.05,32.38 40.96,29.53 40.96,24.26 C13.+
  Bottom 0.305: 25.49,47.62 IC1.10 25.49,62.78 v24.77,63.5 | 25.49,47.62 v24.45,47.62 | v49.53,81.6 48.9,81.6 v43.81,76.52 43.81,61.59 | 43.81,61.59 43.81,52.7 45.4,51.12 | 45.4,51.12 48.9,51.12 v49.53,51.75 | 45.4,51.12 46.67,49.85 46.67,47.94 39.05,40.32 v39.05,40.01 35.56,40.01 32.7,42.86 27.62,42.86 25.49,45 25.49,47.62 | v49.21,66.67 48.9,66.67 43.81,61.59
  Bottom 1.016: IC2.OUT 36.2,5.08 D1.A C15.1 39.37,10.16 41.59,10.16 C13.+ | v39.05,32.38 v39.05,40.01
/RES  (via drill 0.6)
  Top 0.305: S2.3 31.83,44.77 | 31.83,44.77 28.89,44.77 JP3.1 26.04,44.77 23.39,44.77 arc90 R1.1 23.18,43.81 23.13,43.77 C4.2 | v36.83,52.7 36.83,52.39 35.56,51.12 35.56,46.99 33.34,44.77 31.83,44.77
  Bottom 0.305: IC1.30 36.7,52.58 v36.83,52.7
DERE0  (via drill 0.6)
  Top 0.305: v44.13,79.69 44.88,79.69 IC9.3 IC9.2
  Bottom 0.305: IC1.6 23.49,64.13 39.37,79.69 v44.13,79.69
DERE1  (via drill 0.6)
  Top 0.305: v43.81,49.21 IC5.3 IC5.2
  Bottom 0.305: IC1.47 41.22,44.08 43.81,46.67 v43.81,49.21
DERE2  (via drill 0.6)
  Top 0.305: v31.75,64.14 IC10.3 IC10.2
  Bottom 0.305: IC1.16 28.49,60.87 v31.75,64.14
DERE3  (via drill 0.6)
  Top 0.305: v24.77,38.73 26.04,40.01 32.7,40.01 33.97,38.73 IC11.2 IC11.3
  Bottom 0.305: IC1.67 24.99,38.96 v24.77,38.73
ENT  (via drill 0.6)
  Top 0.305: 24.13,90.7 34.61,90.7 C23.1 38.42,92.39 FERITE.2 | 24.13,90.7 R11.1 arc90 18.95,90.81 12.38,90.81 11.11,89.53 11.11,87 12.38,85.72 U$1.3 18.1,85.72 18.31,85.51 R12.1 | v24.13,90.81 24.13,90.7
  Bottom 0.305: FX1.7 v24.13,90.81
ETH  (via drill 0.6)
  Top 0.305: v33.66,68.26 33.66,73.34 37.15,76.83 IC4.9
  Bottom 0.305: IC1.19 29.99,60.78 33.66,64.45 v33.66,68.26
GND  (via drill 0.6)
  Top 0.305: 34.61,54.93 v26.67,54.93 22.54,54.93 22.23,54.61 v22.23,53.98 JP3.6 | 34.61,54.93 34.61,51.12 Q3.2 29.84,51.12 29.84,47.34 S2.1 31.83,47.62 | v26.99,63.5 26.99,62.27 C26.2 | IC11.5 42.23,36.2 45.09,41.59 DMX4IN.2 | IC4.2 40.96,67.94 v42.55,69.53 44.45,71.44 | 44.45,71.44 DMX3IN.2 | 36.83,86.36 37.05,86.58 R8.1 C22.2 43.71,86.36 DMX1IN.2 | 36.83,86.36 36.83,83.19 35.56,83.19 35.56,79.38 IC4.11 40.42,79.38 arc-90 C25.1 41.59,78.21 41.59,74.93 44.45,71.44 | 36.83,86.36 36.62,86.58 C24.1 35.46,86.68 32.38,86.68 32.38,80.96 30.8,79.38 IC4.18 v27.62,79.38 C18.1 | C23.2 C27.2 | 36.83,87.95 36.83,86.36 | DMX4OUT.2 51.44,41.59 52.39,42.55 52.39,47.31 51.75,47.94 IC5.5 | DMX2IN.2 v42.55,56.52 39.37,56.52 | 39.37,56.52 C21.- | 34.61,54.93 36.2,56.52 39.37,56.52 | IC9.5 51.75,77.79 52.39,77.15 52.39,72.39 51.44,71.44 DMX3OUT.2 | IC10.5 51.75,62.87 52.39,62.23 52.39,57.47 51.44,56.52 DMX2OUT.2 | C17.1 IC4.22 IC4.21 arc-90 29.4,75.25 v23.5,75.25
  Bottom 0.305: v26.67,54.93 25.99,54.93 IC1.11 25.99,62.82 v26.99,63.5 | IC1.99 22.23,54.08 v22.23,53.98 | DMX4IN.2 DMX4OUT.2 | DMX2IN.2 DMX2OUT.2 | DMX3IN.2 DMX3OUT.2 | DMX1IN.2 DMX1OUT.2 | v23.5,75.25 23.5,76.94 arc-90 25.93,79.38 v27.62,79.38 | U$1.GND2 4.04,76.07 U$1.LED2.2
  Bottom 1.016: v42.55,69.53 v42.55,56.52 | D4.A 23.5,2.22 31.11,2.22 IC2.GND | U$1.GND1 U$1.GND2
  pour Bottom (isolate 0.61): 54,29 54,0 0,0 0,29
  pour Top: 0,100.01 0.32,28.89 53.98,28.89 53.98,99.69
  pour Bottom: 0.32,100.01 0.32,28.57 53.98,28.89 53.98,100.33
INT  (via drill 0.6)
  Top 0.305: v22.54,65.41 30.8,65.41 32.38,66.99 33.97,66.99 37.47,70.48 IC4.4
  Bottom 0.305: IC1.4 22.49,65.35 v22.54,65.41
MISO  (via drill 0.6)
  Top 0.305: v29.53,52.7 JP3.5 | v36.51,72.71 36.83,73.03 IC4.6
  Bottom 0.305: v29.53,52.7 31.49,52.7 IC1.22 31.49,59.11 36.51,63.82 v36.51,72.71
MOSI  (via drill 0.6)
  Top 0.305: v28.89,48.9 23.5,48.9 JP3.4 | v35.56,70.8 35.56,73.34 36.51,74.3 IC4.7
  Bottom 0.305: v28.89,48.9 28.89,51.44 28.26,52.07 28.26,53.66 30.99,53.66 IC1.21 30.99,59.56 35.56,64.14 v35.56,70.8
N$1  (via drill 0.6)
  Top 0.305: v33.34,49.85 31.75,49.85 Q3.3
  Bottom 0.305: IC1.34 33.34,50.58 v33.34,49.85
N$2  (via drill 0.6)
  Top 0.305: v33.34,53.34 31.75,53.34 Q3.1
  Bottom 0.305: IC1.33 33.34,51.08 v33.34,53.34
N$3
  Bottom 0.305: IC1.51 32.99,39.97 33.02,40.01 33.02,33.97 30.8,31.75 12.38,31.75 3.49,39.05 3.49,61.91 SW1.20
N$4
  Bottom 1.016: R4.2 19.37,19.05 LED1.K
N$5
  Bottom 0.305: IC1.52 32.49,34.39 30.48,32.38 12.7,32.38 4.13,39.37 4.13,59.37 SW1.19
N$6
  Bottom 1.016: F1.2 D3.A
N$7
  Bottom 0.305: IC1.53 31.99,34.84 30.16,33.02 13.02,33.02 4.76,39.69 4.76,56.83 SW1.18
N$8
  Top 0.305: R7.1 2.01,80.64 U$1.LED2.1
N$9
  Bottom 0.305: IC1.54 31.49,35.3 29.84,33.66 13.02,33.66 5.71,39.69 5.71,54.29 SW1.17
N$10
  Bottom 1.016: X1.1 12.53,13.51 F1.1
N$11
  Top 0.305: IC4.27 16.19,67.94 16.19,75.25 6.67,81.92 R7.2
N$12
  Bottom 1.016: R2.2 26.04,22.23 IC3.1 25.72,22.23 23.5,20 R3.1
N$13
  Top 0.305: IC4.26 17.14,69.22 17.14,75.88 R6.2
N$14
  Top 0.305: R6.1 2.01,86.89 1.59,87.31 1.59,89.12 U$1.LED1.1
N$15
  Top 0.305: R13.2 50.16,60.22 DMX2OUT.1 49.53,59.05 48.26,57.78 48.26,55.24 | DMX2IN.1 46.99,53.98 48.26,55.24 | IC5.7 48.9,50.48 48.26,51.12 48.26,55.24
N$16
  Top 0.305: DMX2IN.3 46.04,59.91 R13.1 | IC5.6 51.75,49.21 52.39,49.85 52.39,53.34 51.59,54.13 50.32,54.13 DMX2OUT.3
  Bottom 0.305: DMX2IN.3 46.99,59.05 49.21,61.28 51.12,61.28 52.39,60.01 52.39,54.93 51.44,53.98 DMX2OUT.3
N$17
  Top 0.305: DMX1IN.3 46.04,90.07 R15.1 | IC9.6 51.75,79.06 52.39,79.69 52.39,82.87 51.44,83.82 DMX1OUT.3
  Bottom 0.305: DMX1IN.3 46.67,88.9 48.9,91.12 51.44,91.12 52.39,90.17 52.39,85.72 51.12,83.82 DMX1OUT.3
N$18
  Top 0.305: R14.2 50.16,75.14 DMX3OUT.1 49.21,73.98 48.26,73.03 48.26,70.48 48.26,70.17 | DMX3IN.1 46.99,68.9 48.26,70.17 | IC10.7 48.9,65.41 48.26,66.04 48.26,70.17
N$19
  Top 0.305: DMX3IN.3 46.04,74.83 R14.1 | IC10.6 51.75,64.14 52.39,64.77 52.39,68.26 51.59,69.06 50.32,69.06 DMX3OUT.3
  Bottom 0.305: DMX3IN.3 46.99,73.98 49.21,76.2 51.12,76.2 52.39,74.93 52.39,69.85 51.44,68.9 DMX3OUT.3
N$20
  Top 0.305: C18.2 23.91,78.74 Q2.2 20,78.74 20,70.17 27.3,70.17 28.89,71.75 IC4.24
N$21
  Top 0.305: IC4.23 C17.2 arc-90 26.89,72.07 21.91,72.07 Q2.1
N$26
  Top 0.305: R8.2 38.1,83.95 IC4.14
N$27  (via drill 0.6)
  Top 0.305: IC4.1 v40.96,66.67 | v40.96,60.96 C21.+
  Bottom 0.305: v40.96,66.67 v40.96,60.96
N$28
  Top 0.305: IC11.7 38.73,38.73 38.73,35.56 39.37,34.92 42.86,34.92 DMX4IN.1 46.99,39.05 48.26,40.32 48.26,42.86 49.53,44.13 DMX4OUT.1 50.16,45.3 R16.2
N$29
  Top 0.305: R10.1 42.44,82.66 R9.1 41.7,84.88 C22.1
N$30  (via drill 0.6)
  Top 0.305: C24.2 34.92,84.14 v34.92,78.11 IC4.10 | R5.1 25.5,78.11 v27.3,78.11
  Bottom 0.305: v34.92,78.11 v27.3,78.11
N$31
  Top 0.305: R15.2 50.16,89.75 DMX1OUT.1 49.21,88.9 48.26,87.95 48.26,85.41 48.26,85.09 | DMX1IN.1 46.67,83.82 48.26,85.09 | IC9.7 48.9,80.33 48.26,80.96 48.26,85.09
N$32
  Top 0.305: IC11.6 42.23,37.78 43.5,41.27 43.81,42.55 44.45,44.13 DMX4IN.3 46.04,44.98 R16.1
  Bottom 0.305: DMX4IN.3 46.99,44.13 49.21,46.35 51.12,46.35 52.39,45.09 52.39,40.01 51.44,39.05 DMX4OUT.3
N$33  (via drill 0.6)
  Top 0.305: v17.14,96.2 v13.34,96.2
  Bottom 0.305: FX1.11 25.4,96.2 v17.14,96.2 | v13.34,96.2 J1.1
N$34
  Bottom 0.305: FX1.9 15.88,97.79 J1.2
N$35  (via drill 0.6)
  Top 0.305: v19.05,93.98 v14.61,93.98
  Bottom 0.305: FX1.16 31.75,93.98 v19.05,93.98 | v14.61,93.98 14.61,85.72 J1.3
N$36
  Bottom 0.305: FX1.14 29.21,95.57 18.1,95.57 18.1,94.93 17.14,94.93 17.14,81.92 J1.6
N$37
  Bottom 0.305: IC1.90 16.14,49.58 JP2.4
N$38
  Bottom 0.305: IC1.91 16.6,50.08 14.92,51.75 14.92,53.34 JP2.3
N$39
  Bottom 0.305: IC1.92 17.05,50.58 15.56,52.07 15.56,55.24 JP2.2
N$40
  Bottom 0.305: IC1.93 17.5,51.08 16.19,52.39 16.19,57.15 JP2.1
N$41
  Bottom 0.305: IC1.43 36.55,46.08 JP1.1
N$42
  Bottom 0.305: IC1.44 37.01,45.58 40.01,46.99 JP1.2
N$43
  Bottom 0.305: FX1.10 24.13,99.06 15.24,99.06 13.97,98.42 C2.1
N$44
  Bottom 0.305: FX1.15 30.48,99.06 33.66,99.06 C1.1
N$250
  Bottom 1.016: LED1.A 14.48,20.77 14.48,20.95 14.61,20.95 | IC2.IN 26.67,7.62 26.35,7.3 | 26.35,7.3 26.04,6.99 D1.C | 23.5,10.16 D4.C 22.86,12.06 D3.C 19.68,15.24 14.61,15.24 LED1.A | 23.5,10.16 26.35,7.3 | C16.1 14.61,20.95 | LED1.A 14.61,20.95 | C11.+ 17.78,4.45 23.5,10.16
RXD1  (via drill 0.6)
  Top 0.305: v40.32,45.72 43.81,45.72 45.4,47.31 45.4,47.84 IC5.4
  Bottom 0.305: IC1.45 39.68,45.08 v40.32,45.72
RXD2  (via drill 0.6)
  Top 0.305: v26.99,59.37 34.29,59.37 37.78,62.87 IC10.4
  Bottom 0.305: IC1.12 26.49,58.87 v26.99,59.37
RXD3  (via drill 0.6)
  Top 0.305: v27.62,38.73 30.16,36.2 IC11.4
  Bottom 0.305: 26.99,40.64 IC1.63 26.99,39.37 v27.62,38.73
SCK  (via drill 0.6)
  Top 0.305: v27.62,51.12 27.62,50.48 JP3.3 | v34.61,69.53 34.61,73.34 36.83,75.56 IC4.8
  Bottom 0.305: v27.62,51.12 27.62,54.29 30.49,54.29 IC1.20 30.49,60.02 34.61,64.14 v34.61,69.53
SW1_5
  Bottom 0.305: IC1.60 28.49,38.01 27.94,37.47 14.61,37.47 13.65,38.42 13.65,49.21 SW1.16
SW1_6
  Bottom 0.305: IC1.59 28.99,37.56 28.26,36.83 14.61,36.83 13.02,38.1 13.02,46.99 SW1.15
SW1_7
  Bottom 0.305: IC1.58 29.49,37.11 28.57,36.2 14.29,36.2 12.38,37.78 12.38,45.09 SW1.14
SW1_8
  Bottom 0.305: IC1.57 29.99,36.66 28.89,35.56 13.97,35.56 11.75,37.47 11.75,42.86 SW1.13
SW1_9
  Bottom 0.305: IC1.56 30.49,36.2 29.21,34.92 13.65,34.92 11.11,37.15 11.11,41.59 SW1.12
SW1_10
  Bottom 0.305: IC1.55 30.99,35.75 29.53,34.29 13.34,34.29 9.21,37.78 SW1.11
TPIN+  (via drill 0.6)
  Top 0.305: R9.2 40.01,84.14 40.74,83.4 40.74,82.65 40.01,81.92 IC4.13 v36.83,81.92 | v22.86,81.92 22.86,79.69 17.78,79.69 U$1.8 | v21.91,92.39 13.02,92.39 v12.06,93.34
  Bottom 0.305: v36.83,81.92 v22.86,81.92 | FX1.1 31.75,92.39 v21.91,92.39 | v12.06,93.34 12.06,78.74 15.24,78.74 U$1.8
TPIN-  (via drill 0.6)
  Top 0.305: R10.2 42.12,80.64 IC4.12 v36.83,80.64 | v21.91,80.64 U$1.7
  Bottom 0.305: v36.83,80.64 v21.91,80.64 | FX1.3 29.21,87.31 27.3,87.31 25.72,85.72 18.41,85.72 18.41,80.64 U$1.7
TPOUT+  (via drill 0.6)
  Top 0.305: IC4.17 30.8,80.64 31.75,81.6 31.75,87 29.84,88.9 FX1.6 | FX1.6 19.15,88.9 R11.2 14.07,89 U$1.1 | v25.4,87.63 FX1.6
  Bottom 0.305: FX1.6 v25.4,87.63
TPOUT-  (via drill 0.6)
  Top 0.305: U$1.2 16.09,87.21 R12.2 21.91,87.21 v22.01,87.21 27.3,81.92 IC4.16
  Bottom 0.305: FX1.8 22.01,88.9 v22.01,87.21
TXD0  (via drill 0.6)
  Top 0.305: v44.13,81.6 IC9.1
  Bottom 0.305: IC1.3 21.91,64.45 21.91,64.77 19.45,67.39 19.45,84.53 41.59,84.45 v44.13,81.6
TXD1  (via drill 0.6)
  Top 0.305: v42.86,51.75 IC5.1
  Bottom 0.305: IC1.46 40.77,44.58 42.86,46.67 v42.86,51.75
TXD2  (via drill 0.6)
  Top 0.305: v32.7,65.41 43.5,65.41 44.77,66.67 IC10.1
  Bottom 0.305: IC1.13 26.99,58.42 27.3,58.42 arc90 27.94,59.05 27.94,59.69 arc90 27.3,60.33 26.99,60.33 26.99,61.59 30.8,65.41 v32.7,65.41
TXD3  (via drill 0.6)
  Top 0.305: v26.04,38.73 29.53,35.24 36.83,35.24 37.47,35.88 37.47,39.37 36.83,40.01 IC11.1
  Bottom 0.305: IC1.64 26.49,39.19 v26.04,38.73
VCC
  Bottom 1.016: IC3.3 33.02,20.32 D2.C
(copper drawn outside any net)
  shapes: Top area x2

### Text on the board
Bottom: Original U.Radig | Modified T.Halenka | and H.D. Tech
